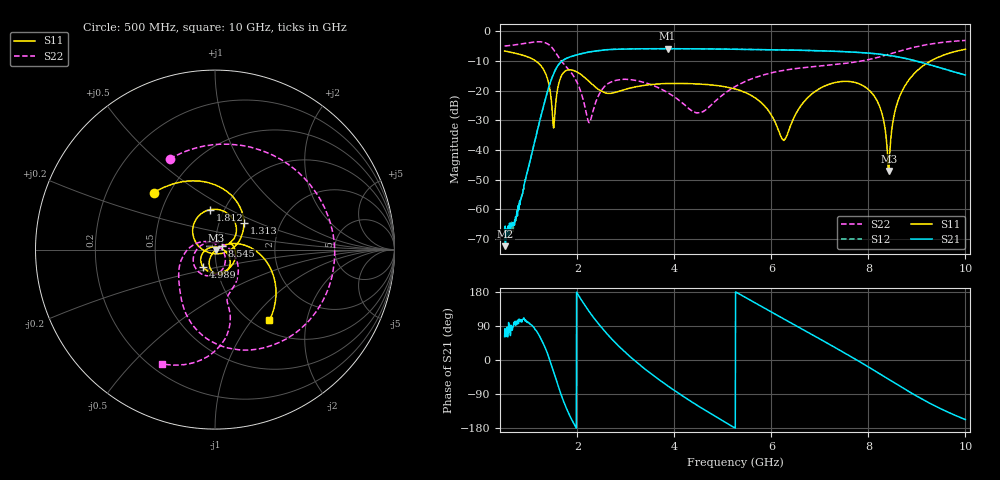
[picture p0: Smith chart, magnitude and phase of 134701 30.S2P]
!  2-Port S-parameters saved by WinCal
! VAR MeasName=S-Parameters (CALIBRATED_DATA) read from VNA (N5242A)
! VAR MeasDate=2013-7-3 16:33:11
! VAR NAME=134701 30
! VAR FILENAME=134701 30.S2P
! VAR DATE=2013-7-3 16:33:11
! VAR PHYS_PORTS=1,2
# Hz S MA R 50
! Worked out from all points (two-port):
!   1601 points, 500 MHz to 10 GHz, reference 50 ohm
!   highest |S21| = -5.86 dB at 3.861 GHz (marker M1); lowest = -72.5 dB at 517.8 MHz (marker M2)
!   |S21| within 3 dB of the highest: 1.813 GHz to 8.678 GHz (6.865 GHz wide, 131 % of centre)
!   lowest |S11| = -47.1 dB at 8.421 GHz (marker M3), VSWR 1.01, Z = 50.4 - j0.238 ohm
!   |S11| at or under -10 dB: 1.142 GHz to 9.285 GHz (8.143 GHz wide, 156 % of centre)
!   |S22| runs from -30.8 to -3.1 dB; largest |S21 - S12| = 0.0019
!   S11 on the Smith chart (normalised r, x): 500 MHz: 0.41, +0.34; 1.313 GHz: 1.31, +0.41; 1.812 GHz: 0.86, +0.40; 4.989 GHz: 0.86, -0.17; 8.545 GHz: 1.08, +0.04; 10 GHz: 1.17, -1.23
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5e8  0.4654 136.9  0.0003258 61.5  0.0004854 67.9  0.5645 116.5
5.178125e8  0.4625 135.5  0.000238 64.9  0.0002383 84.2  0.5663 114.1
9.15625e8  0.3857 100.4  0.002825 107.1  0.002835 107.0  0.6264 49.4
1.313438e9  0.2189 42.7  0.05927 39.1  0.05963 39.0  0.6504 -42.2
1.509375e9  0.0235 -90.6  0.1912 -30.3  0.191 -30.4  0.4911 -96.6
1.812188e9  0.2244 97.2  0.3602 -138.4  0.36 -138.4  0.232 -150.1
2.085312e9  0.1844 51.9  0.4203 157.8  0.4203 157.9  0.08776 150.7
2.251562e9  0.1408 35.2  0.4489 126.4  0.4486 126.4  0.02901 46.2
2.601875e9  0.09054 24.8  0.4883 70.4  0.4894 70.4  0.126 -75.4
3.670625e9  0.1297 -47.6  0.509 -50.7  0.5084 -50.7  0.1118 -172.7
3.860625e9  0.1318 -61.6  0.5091 -68.0  0.5095 -68.1  0.09273 173.2
4.478125e9  0.1293 -98.2  0.5055 -120.2  0.5067 -120.2  0.04202 84.0
4.98875e9  0.1182 -123.3  0.501 -159.9  0.5016 -159.9  0.08361 0.6
5.25e9  0.1066 -136.6  0.4975 -179.4  0.498 -179.4  0.1167 -18.2
6.253438e9  0.01466 89.2  0.4843 108.5  0.4845 108.5  0.2192 -58.5
6.835312e9  0.08768 -26.6  0.4729 67.1  0.4734 67.1  0.2518 -70.8
7.975312e9  0.1088 -104.4  0.4302 -16.4  0.4304 -16.5  0.3295 -76.6
8.254375e9  0.04801 -121.8  0.4087 -38.2  0.4091 -38.3  0.3741 -76.9
8.420625e9  0.004408 -32.4  0.3926 -51.2  0.3916 -51.3  0.4084 -78.1
8.545312e9  0.04363 27.2  0.3777 -60.9  0.3775 -61.1  0.4382 -79.5
9.014375e9  0.2199 -0.5  0.3114 -96.7  0.3105 -96.7  0.554 -88.8
1e10  0.4978 -52.5  0.1831 -157.3  0.1831 -157.2  0.7005 -114.7
